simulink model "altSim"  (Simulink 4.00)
settings: Solver=FixedStepDiscrete  StartTime=0.0  StopTime=2  RelTol=1e-3

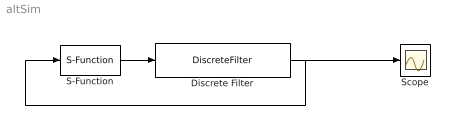
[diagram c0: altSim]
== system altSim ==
  Discrete Filter : DiscreteFilter  Numerator=[0.014216]  Denominator=[1 -1.87036 0.884513]  SampleTime=1/1024  Realization=auto
  S-Function : S-Function  FunctionName=altSim  Parameters=nodeName, nodeNumber  PortCounts=[]  SFunctionModules=''  mask{nodeName='127.0.0.1', nodeNumber=1}
      mask prompts: nodeName "Node name"; nodeNumber "Node number"
  Scope : Scope
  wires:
  Discrete Filter/1 -> S-Function/1, Scope/1
  S-Function/1 -> Discrete Filter/1
